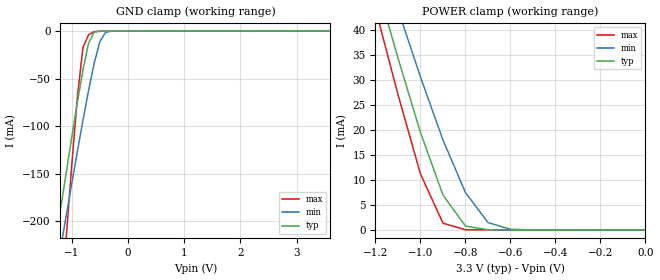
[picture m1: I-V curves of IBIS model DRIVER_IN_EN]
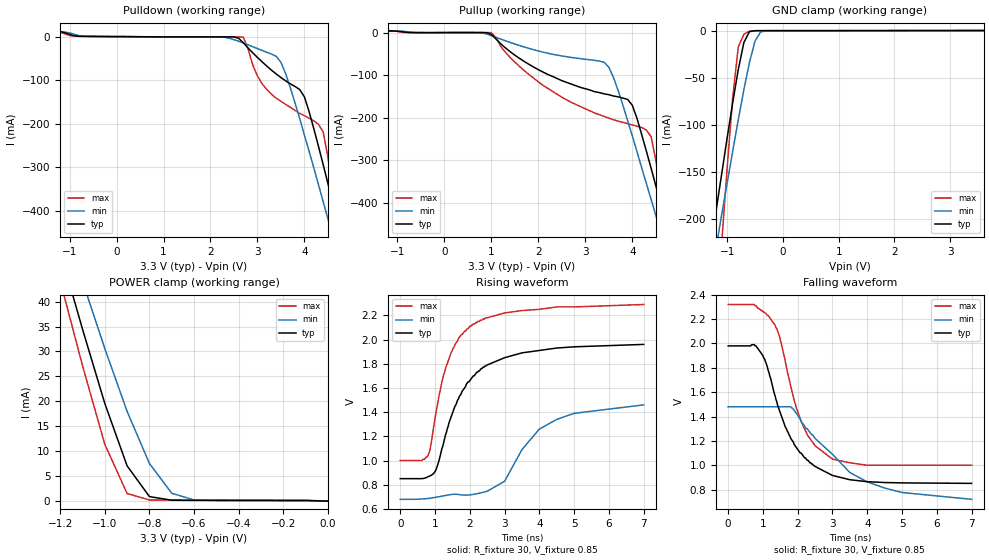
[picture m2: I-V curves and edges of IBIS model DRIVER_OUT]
|   Texas Instruments Incorporated
|   Data Transmissions Products
|   IBIS Model for TB5D2H
|   16DW SOIC Package
[IBIS Ver]   3.2
[Comment char]   |_char
[File name]   tb5d2hdw_3v.ibs
[File Rev]   1.0
[Date]   23Jan04
[Source]   File originated at Texas Instruments Incorporated.
   Data Transmission Products Group. All data based on
   Simulation.
[Notes]
[Disclaimer]
(C) Copyright Texas Instruments Incorporated 2004
   All rights reserved
  Texas Instruments Incorporated hereby grants the user of this IBIS
model a non-exclusive, nontransferable license to use this IBIS model
under the following terms.  Before using this IBIS model, the user
should read this license.  If the user does not accept these terms,
the IBIS model should be returned to Texas Instruments within 30 days.
  The user is granted this license only to use the IBIS model and
is not granted rights to sell, load, rent, lease or license the IBIS
model in whole or in part, or in modified form to anyone other than
user.  User may modify the IBIS model to suit its specific applications
but rights to derivative works and such modifications shall belong to
Texas Instruments.
  This IBIS model is provided on an "AS IS" basis and Texas Instruments
makes absolutely no warranty with respect to the information contained
herein.  TEXAS INSTRUMENTS DISCLAIMS AND CUSTOMER WAIVES ALL WARRANTIES,
EXPRESS OR IMPLIED, INCLUDING WARRANTIES OF MERCHANTABILITY OR FITNESS
FOR A PARTICULAR PURPOSE. The entire risk as to quality and performance
is with the Customer. ACCORDINGLY, IN NO EVENT SHALL THE COMPANY BE LIABLE
FOR ANY DAMAGES, WHETHER IN CONTRACT OR TORT,INCLUDING ANY LOST PROFITS
OR OTHER INCIDENTAL, CONSEQUENTIAL, EXEMPLARY, OR PUNITIVE DAMAGES ARISING
OUT OF THE USE OR APPLICATION OF THE IBIS model provided in this package.
Further, Texas Instruments reserves the right to discontinue or make changes
without notice to any product herein to improve reliability, function, or
design. Texas Instruments does not convey any license under patent rights
or any other intellectual property rights, including those of third parties.
Contact Texas Instruments at ATTN:DATA TRANSMISSIONS
[Copyright]   Copyright 2004 Texas Instruments, All Rights Reserved
[Component]   TB5D1M
[Manufacturer]  Texas Instruments
[Package]
|   typ   min   max
R_pkg   0.046   0.034   0.057
L_pkg   4.858nH   3.987nH   6.214nH
C_pkg   0.715pF   0.502pF   1.046pF
[Pin]   signal_name   model_name   R_pin   L_pin   C_pin
1   AI   DRIVER_IN_EN   0.057   6.214nH   1.026pF
2   AO   DRIVER_OUT   0.055   5.236nH   0.818pF
3   AO(-)   DRIVER_OUT   0.034   3.987nH   0.723pF
4   E1   DRIVER_IN_EN   0.036   3.996nH   0.726pF
5   BO(-)   DRIVER_OUT   0.036   3.996nH   0.726pF
6   BO   DRIVER_OUT   0.034   3.987nH   0.704pF
7   BI   DRIVER_IN_EN   0.055   5.236nH   0.818pF
8   GND   GND   0.057   6.214nH   1.046pF
9   CI   DRIVER_IN_EN   0.057   6.214nH   0.827pF
10   CO   DRIVER_OUT   0.055   5.236nH   0.597pF
11   CO(-)   DRIVER_OUT   0.034   3.987nH   0.502pF
12   E2   DRIVER_IN_EN   0.036   3.996nH   0.505pF
13   DO(-)   DRIVER_OUT   0.036   3.996nH   0.505pF
14   DO   DRIVER_OUT   0.034   3.987nH   0.502pF
15   DI   DRIVER_IN_EN   0.055   5.236nH   0.597pF
16   VCC   POWER   0.057   6.214nH   0.827pF
[Diff_pin]   inv_pin   vdiff   tdelay_typ   tdelay_min   tdelay_max
| The 'AO(+) (or 'xO(+)')' and inv_pins, 'AO(-) (or 'xO(-)')', pins
| are Diff_pins
   2   3   NA   0   0   0
   6   5   NA   0   0   0
   10   11   NA   0   0   0
   14   13   NA   0   0   0
| Models and submodels in the file (2): DRIVER_IN_EN (Input), DRIVER_OUT (Output_ECL)
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|   Driver Input Model
[Model]   DRIVER_IN_EN
Model_type   Input
|Signals   AI,BI,CI,DI,E1,E2
Vinh = 2.4
Vinl = 0.4
|   typ   min   max
C_comp   964fF   924fF   1010fF
|   typ   min   max
[Temperature Range]   25   -40   125
[Voltage range]   3.3V   3.0V   3.6V
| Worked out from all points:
|   GND clamp passes 1 mA (typ) near -0.59 V on its own axis
|   POWER clamp passes 1 mA (typ) near -0.80 V on its own axis
[GND_clamp]
| Voltage   I(typ)   I(min)   I(max)
-3.6V     -1.15A     -1.09A     -2.3A
-1.3V     -227mA     -264mA     -379mA
-1.2V     -188mA     -230mA     -299mA
-1.1V     -150mA     -195mA     -219mA
-900mV    -75.2mA    -127mA     -70mA
-800mV    -40.9mA    -94mA      -17.2mA
-700mV    -12.7mA    -62.5mA    -3.95mA
-600mV    -1.08mA    -33.7mA    -639uA
-500mV    -134uA     -11.2mA    -147uA
-400mV    -93.8uA    -1.45mA    -117uA
-300mV    -89.9uA    -161uA     -113uA
3.6V      8.46uA     8.25uA     9.83uA
[Power_clamp]
| Note that the[POWER_clamp]voltage table is referenced to Vcc
| and is calculated using Vtable=Vcc - Vmeasured.
|   Voltage   I(typ)   I(min)   I(max)
-3.3V     257mA      242mA      268mA
-1.2V     50.1mA     58.1mA     44.2mA
-1.1V     34.4mA     44.1mA     27.1mA
-1V       19.5mA     30.6mA     11.2mA
-900mV    6.98mA     18mA       1.35mA
-800mV    782uA      7.48mA     43.4uA
-700mV    41.1uA     1.49mA     22.7uA
-600mV    16.5uA     134uA      19.3uA
0V        961nA      961nA      405nA
|   Driver Output Model
[Model]   DRIVER_OUT
Model_type   Output_ECL
| Signals   O(+),O(-)
Vmeas = 1.5V   |Reference voltage for timing measurements
Cref = 0pF   |Timing specification test load capacitance value
Rref = 30   |Note: 30 Ohm load; single ended configuration
| variable   typ   min   max
C_comp   970fF   930fF   1010fF
|   typ   min   max
[Temperature Range]   25   -40   125
[Voltage range]   3.3V   3.0V   3.6V
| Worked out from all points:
|   GND clamp passes 1 mA (typ) near -0.60 V on its own axis
|   POWER clamp passes 1 mA (typ) near -0.80 V on its own axis
|   rising waveform, R_fixture 30, V_fixture 0.85: 20-80 % time 1.07ns typ, 1.26ns min, 781ps max; typ from 0.85 V to 1.96 V
|   falling waveform, R_fixture 30, V_fixture 0.85: 20-80 % time 978ps typ, 1.76ns min, 779ps max; typ from 1.98 V to 0.851 V
[Pulldown]
|   Voltage   I(typ)   I(min)   I(max)
-3.3V     13.3mA     11.2mA     14.8mA
2.5V      -136uA     -6.43mA    -47.6nA
2.7V      -13.7mA    -14mA      -904uA
3V        -47.2mA    -26.9mA    -89.9mA
3.5V      -93.4mA    -58.3mA    -148mA
4V        -138mA     -226mA     -181mA
4.4V      -294mA     -379mA     -219mA
4.5V      -337mA     -418mA     -276mA
4.6V      -380mA     -457mA     -352mA
4.7V      -423mA     -497mA     -433mA
4.8V      -467mA     -536mA     -516mA
6.6V      -1.24A     -1.25A     -2.05A
[Pullup]
|   Voltage   I(typ)   I(min)   I(max)
| Note that the[Pullup]voltage table is referenced to Vcc
| and is calculated using Vtable=Vcc - Vmeasured.
-3.3V     4.07mA     3.16mA     4.71mA
1V        -4.62mA    -7.27mA    -284uA
1.4V      -45mA      -23.2mA    -58.5mA
2V        -87.2mA    -43.3mA    -116mA
3.4V      -144mA     -69.9mA    -197mA
3.6V      -149mA     -106mA     -205mA
4V        -171mA     -243mA     -217mA
4.4V      -319mA     -392mA     -245mA
4.6V      -401mA     -468mA     -375mA
4.7V      -443mA     -506mA     -455mA
4.8V      -484mA     -544mA     -537mA
6.6V      -1.24A     -1.25A     -2.04A
[GND_clamp]
|   Voltage   I(typ)   I(min)   I(max)
| Outputs in High Impedance (off)
-3.6V     -1.36A     -1.24A     -2.55A
-1.3V     -232mA     -271mA     -395mA
-1.2V     -192mA     -232mA     -310mA
-1.1V     -153mA     -196mA     -227mA
-1V       -114mA     -162mA     -146mA
-900mV    -76.3mA    -128mA     -70.9mA
-800mV    -41.2mA    -94.5mA    -17.1mA
-700mV    -12.6mA    -62.7mA    -3.83mA
-600mV    -988uA     -33.7mA    -517uA
-500mV    -39.3uA    -11.1mA    -27.9uA
-300mV    -50.5nA    -88.6uA    -11.9nA
3.6V      138uA      118uA      167uA
[Power_clamp]
| Note that the[POWER_clamp]voltage table is referenced to Vcc
| and is calculated using Vtable=Vcc - Vmeasured.
|   Voltage   I(typ)   I(min)   I(max)
-3.3V     259mA      244mA      270mA
-1.2V     50.1mA     58mA       44.2mA
-1.1V     34.5mA     44.1mA     27.2mA
-1V       19.6mA     30.6mA     11.4mA
-900mV    7.08mA     18mA       1.53mA
-800mV    914uA      7.55mA     234uA
-700mV    180uA      1.58mA     211uA
-600mV    153uA      235uA      204uA
-100mV    128uA      97.7uA     174uA
0V        961nA      961nA      961nA
[Ramp]
|   typ   min   max
dV/dt_r   0.774/1069ps   0.858/804ps   0.577/1207ps
dV/dt_f   0.774/979ps   0.859/707ps   0.575/1271ps
R_load = 40ohm
[Rising Waveform]
R_fixture = 30
V_fixture = 0.85
V_fixture_min = 0.65
V_fixture_max = 1.00
C_fixture = 0
|   V(typ)   V(min)   V(max)
0s        850mV      679mV      1V
800ps     866mV      686mV      1.04V
1.025ns   922mV      696mV      1.39V
1.3ns     1.21V      711mV      1.76V
1.675ns   1.51V      719mV      2.01V
2.1ns     1.7V       720mV      2.13V
3ns       1.85V      828mV      2.22V
3.5ns     1.89V      1.09V      2.24V
4.5ns     1.93V      1.34V      2.27V
7ns       1.96V      1.46V      2.29V
[Falling Waveform]
R_fixture = 30
V_fixture = 0.85
V_fixture_min = 0.65
V_fixture_max = 1.00
C_fixture = 0
|   V(typ)   V(min)   V(max)
0s        1.98V      1.48V      2.32V
800ps     1.98V      1.48V      2.31V
1.05ns    1.87V      1.48V      2.25V
1.35ns    1.57V      1.48V      2.15V
1.8ns     1.22V      1.48V      1.65V
2.125ns   1.09V      1.35V      1.34V
3ns       916mV      1.09V      1.05V
3.5ns     881mV      940mV      1.02V
4.5ns     858mV      813mV      1V
7ns       851mV      720mV      1V
